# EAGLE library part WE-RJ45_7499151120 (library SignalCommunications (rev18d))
Order Code 7499151120 Design THT xBase-T 10/100/1000 Base-T Ports 1x2 Stacked Application Standard Tab Position UP & DOWN LED (Left-Right) YELLOW-GREEN EMI Fingers Yes Details see: http://katalog.we-online.de/en/pbs/WE-LAN_RJ45/7499151120? Updated by Yingchun Shan 2016-08-29 2016(C) Würth Elektronik
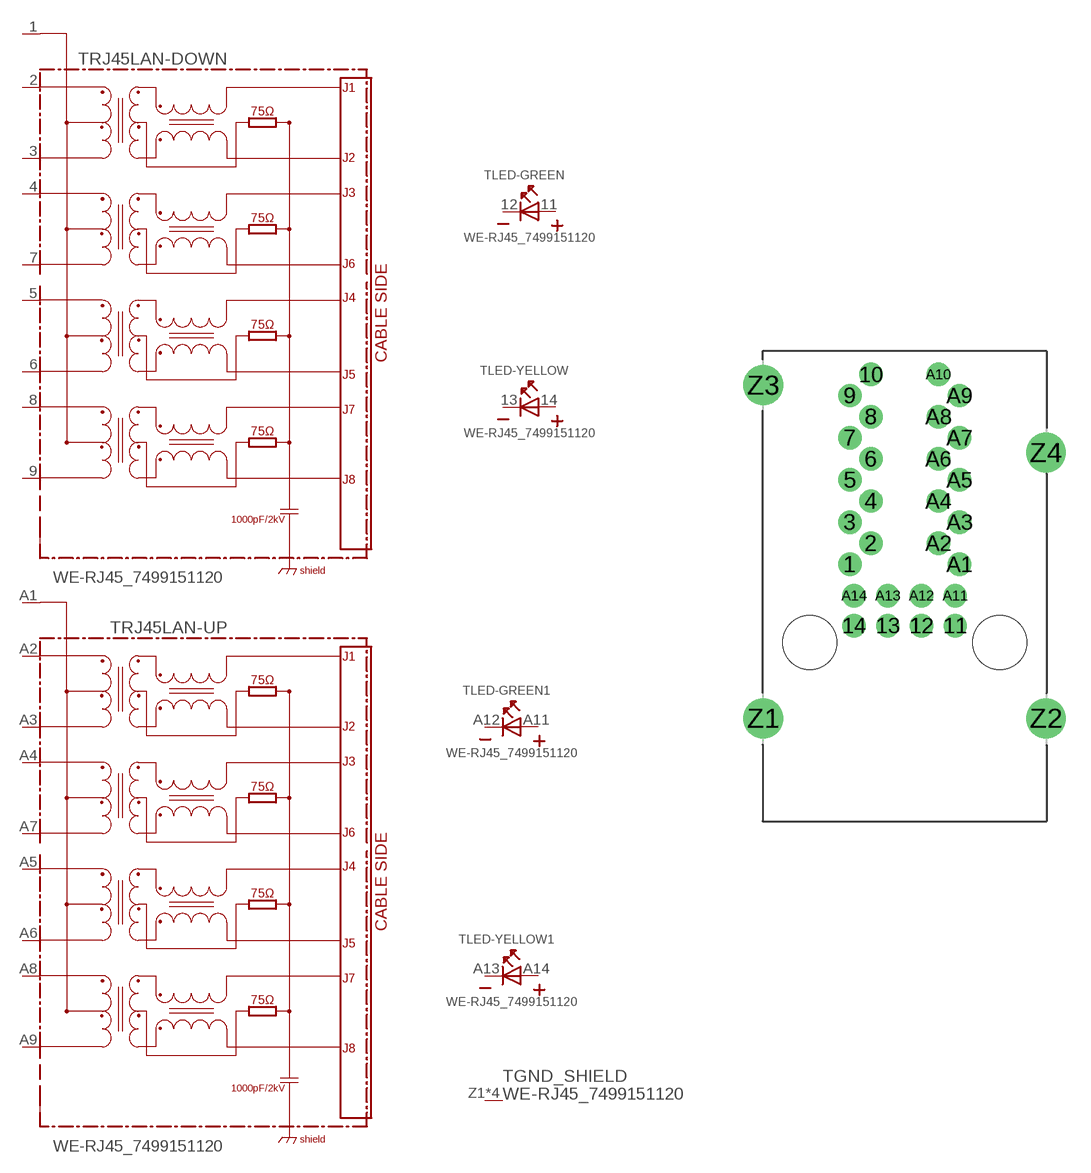
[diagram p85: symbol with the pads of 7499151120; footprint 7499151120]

Designator prefix T; gates RJ45LAN-DOWN=7499151120 RJ45LAN-UP=7499151120 LED-GREEN=LED2PIN LED-YELLOW=LED2PIN LED-GREEN1=LED2PIN LED-YELLOW1=LED2PIN GND_SHIELD=GND_PIN

## WE-RJ45_7499151120 (COMPANY-URL: http://www.we-online.de; CREATED-BY: Christin Zierenner; CREATED-DATE: AUG 2012; DATASHEET-URL: http://katalog.we-online.de/kataloge/eisos/media/pdf/7499151120.pdf; MANUFACTURER: Würth Elektronik eiSos GmbH)  [7499151120]
1  RJ45LAN-DOWN:1
2  RJ45LAN-DOWN:2
3  RJ45LAN-DOWN:3
4  RJ45LAN-DOWN:4
5  RJ45LAN-DOWN:5
6  RJ45LAN-DOWN:6
7  RJ45LAN-DOWN:7
8  RJ45LAN-DOWN:8
9  RJ45LAN-DOWN:9
11  LED-GREEN:A  pas
12  LED-GREEN:K  pas
13  LED-YELLOW:K  pas
14  LED-YELLOW:A  pas
A1  RJ45LAN-UP:1
A2  RJ45LAN-UP:2
A3  RJ45LAN-UP:3
A4  RJ45LAN-UP:4
A5  RJ45LAN-UP:5
A6  RJ45LAN-UP:6
A7  RJ45LAN-UP:7
A8  RJ45LAN-UP:8
A9  RJ45LAN-UP:9
A11  LED-GREEN1:A  pas
A12  LED-GREEN1:K  pas
A13  LED-YELLOW1:K  pas
A14  LED-YELLOW1:A  pas
Z1  GND_SHIELD:1  pwr
Z2  GND_SHIELD:1  pwr
Z3  GND_SHIELD:1  pwr
Z4  GND_SHIELD:1  pwr

## Footprint 7499151120 (pad centres in mm)
MAX HEIGHT=26.0mm PORTS----1X2 LED -YES
drill 0.9: 1 -3.3,4.7; 2 -2.03,5.97; 3 -3.3,7.24; 4 -2.03,8.51; 5 -3.3,9.78; 6 -2.03,11.05; 7 -3.3,12.32; 8 -2.03,13.59; 9 -3.3,14.86; 10 -2.03,16.13; 11 3.045,1.01; 12 1.015,1.01; 13 -1.015,1.01; 14 -3.045,1.01; A1 3.3,4.7; A2 2.03,5.97; A3 3.3,7.24; A4 2.03,8.51; A5 3.3,9.78; A6 2.03,11.05; A7 3.3,12.32; A8 2.03,13.59; A9 3.3,14.86; A10 2.03,16.13; A11 3.045,2.81; A12 1.015,2.81; A13 -1.015,2.81; A14 -3.045,2.81
drill 1.6: Z1 -8.505,-4.57; Z2 8.505,-4.57; Z3 -8.505,15.49; Z4 8.505,11.43
hole 3.25 at 5.715,0
hole 3.25 at -5.715,0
